//{attribute 'qualified_only'}
{attribute 'strict'}
TYPE E_CrossAutomaticActiveState :
(
	eCrossAutoActive_WaitBeforeH	:= 0,
	eCrossAutoActive_ReleaseH		:= 1,
	eCrossAutoActive_WaitBeforeV	:= 2,
	eCrossAutoActive_ReleaseV		:= 3 
);
END_TYPE
